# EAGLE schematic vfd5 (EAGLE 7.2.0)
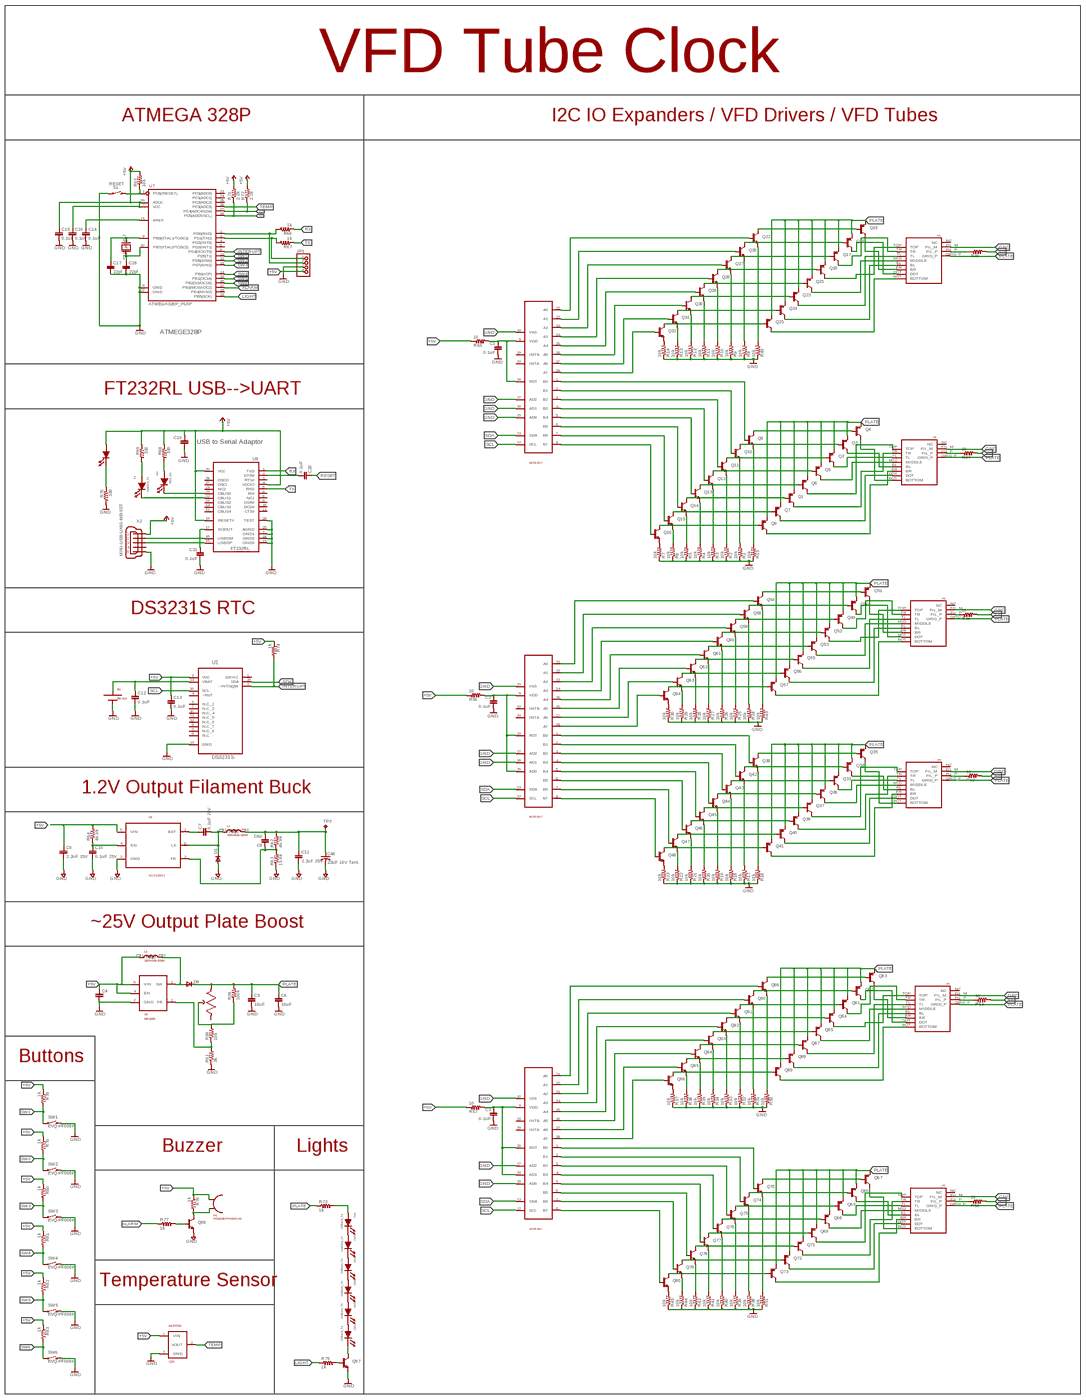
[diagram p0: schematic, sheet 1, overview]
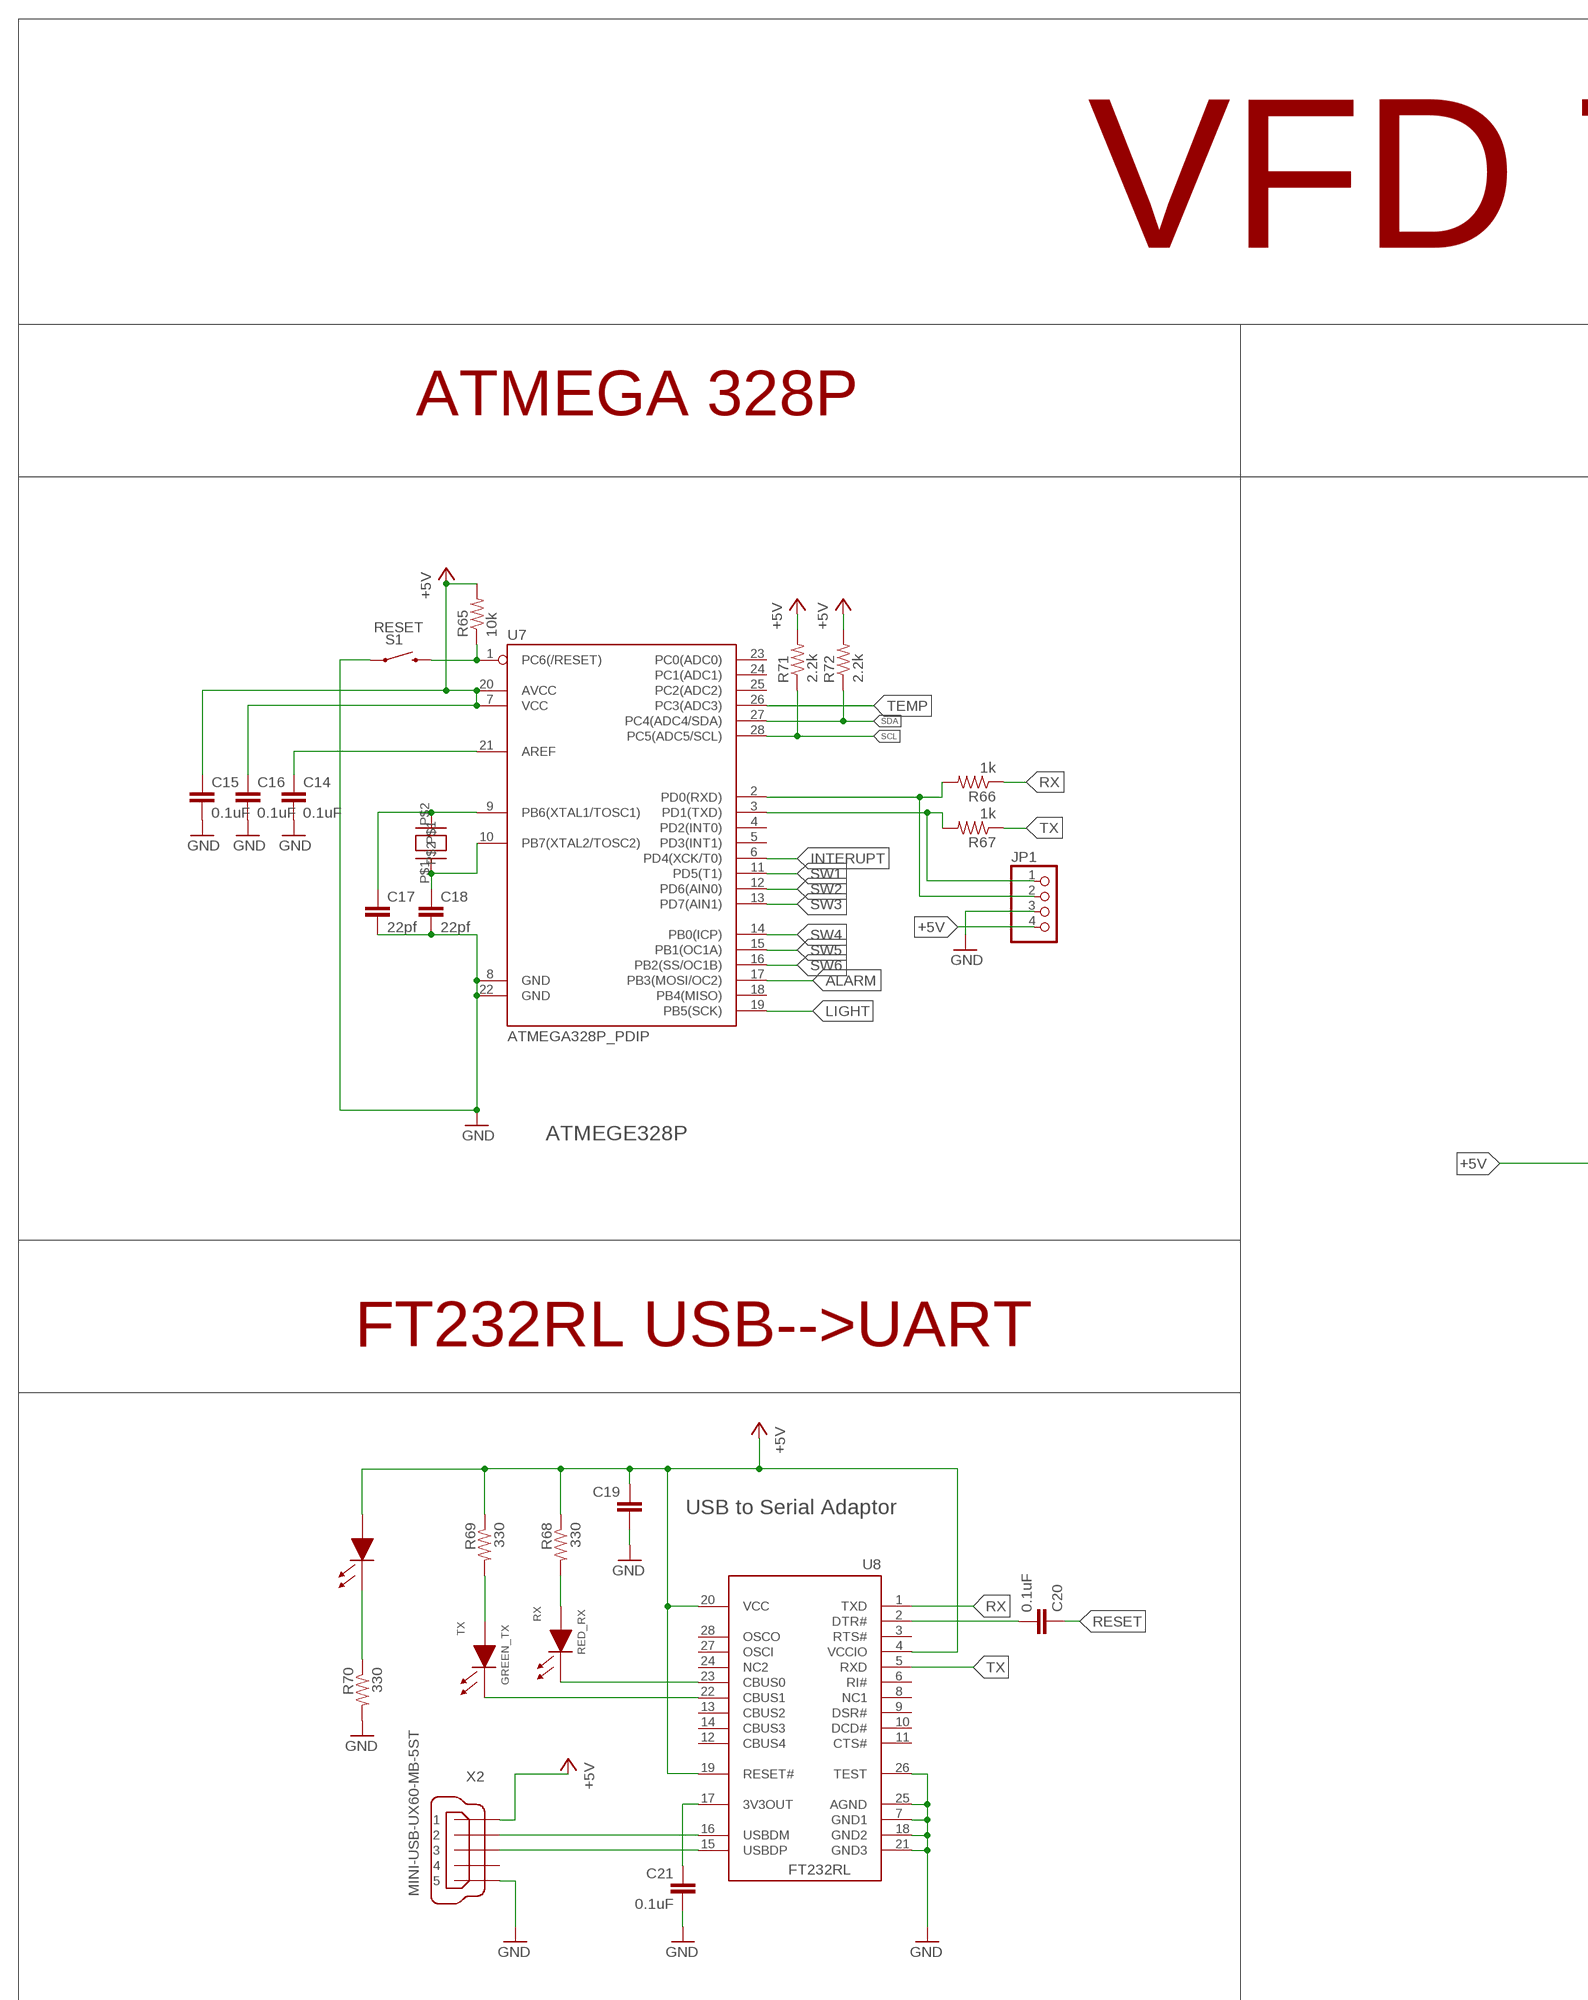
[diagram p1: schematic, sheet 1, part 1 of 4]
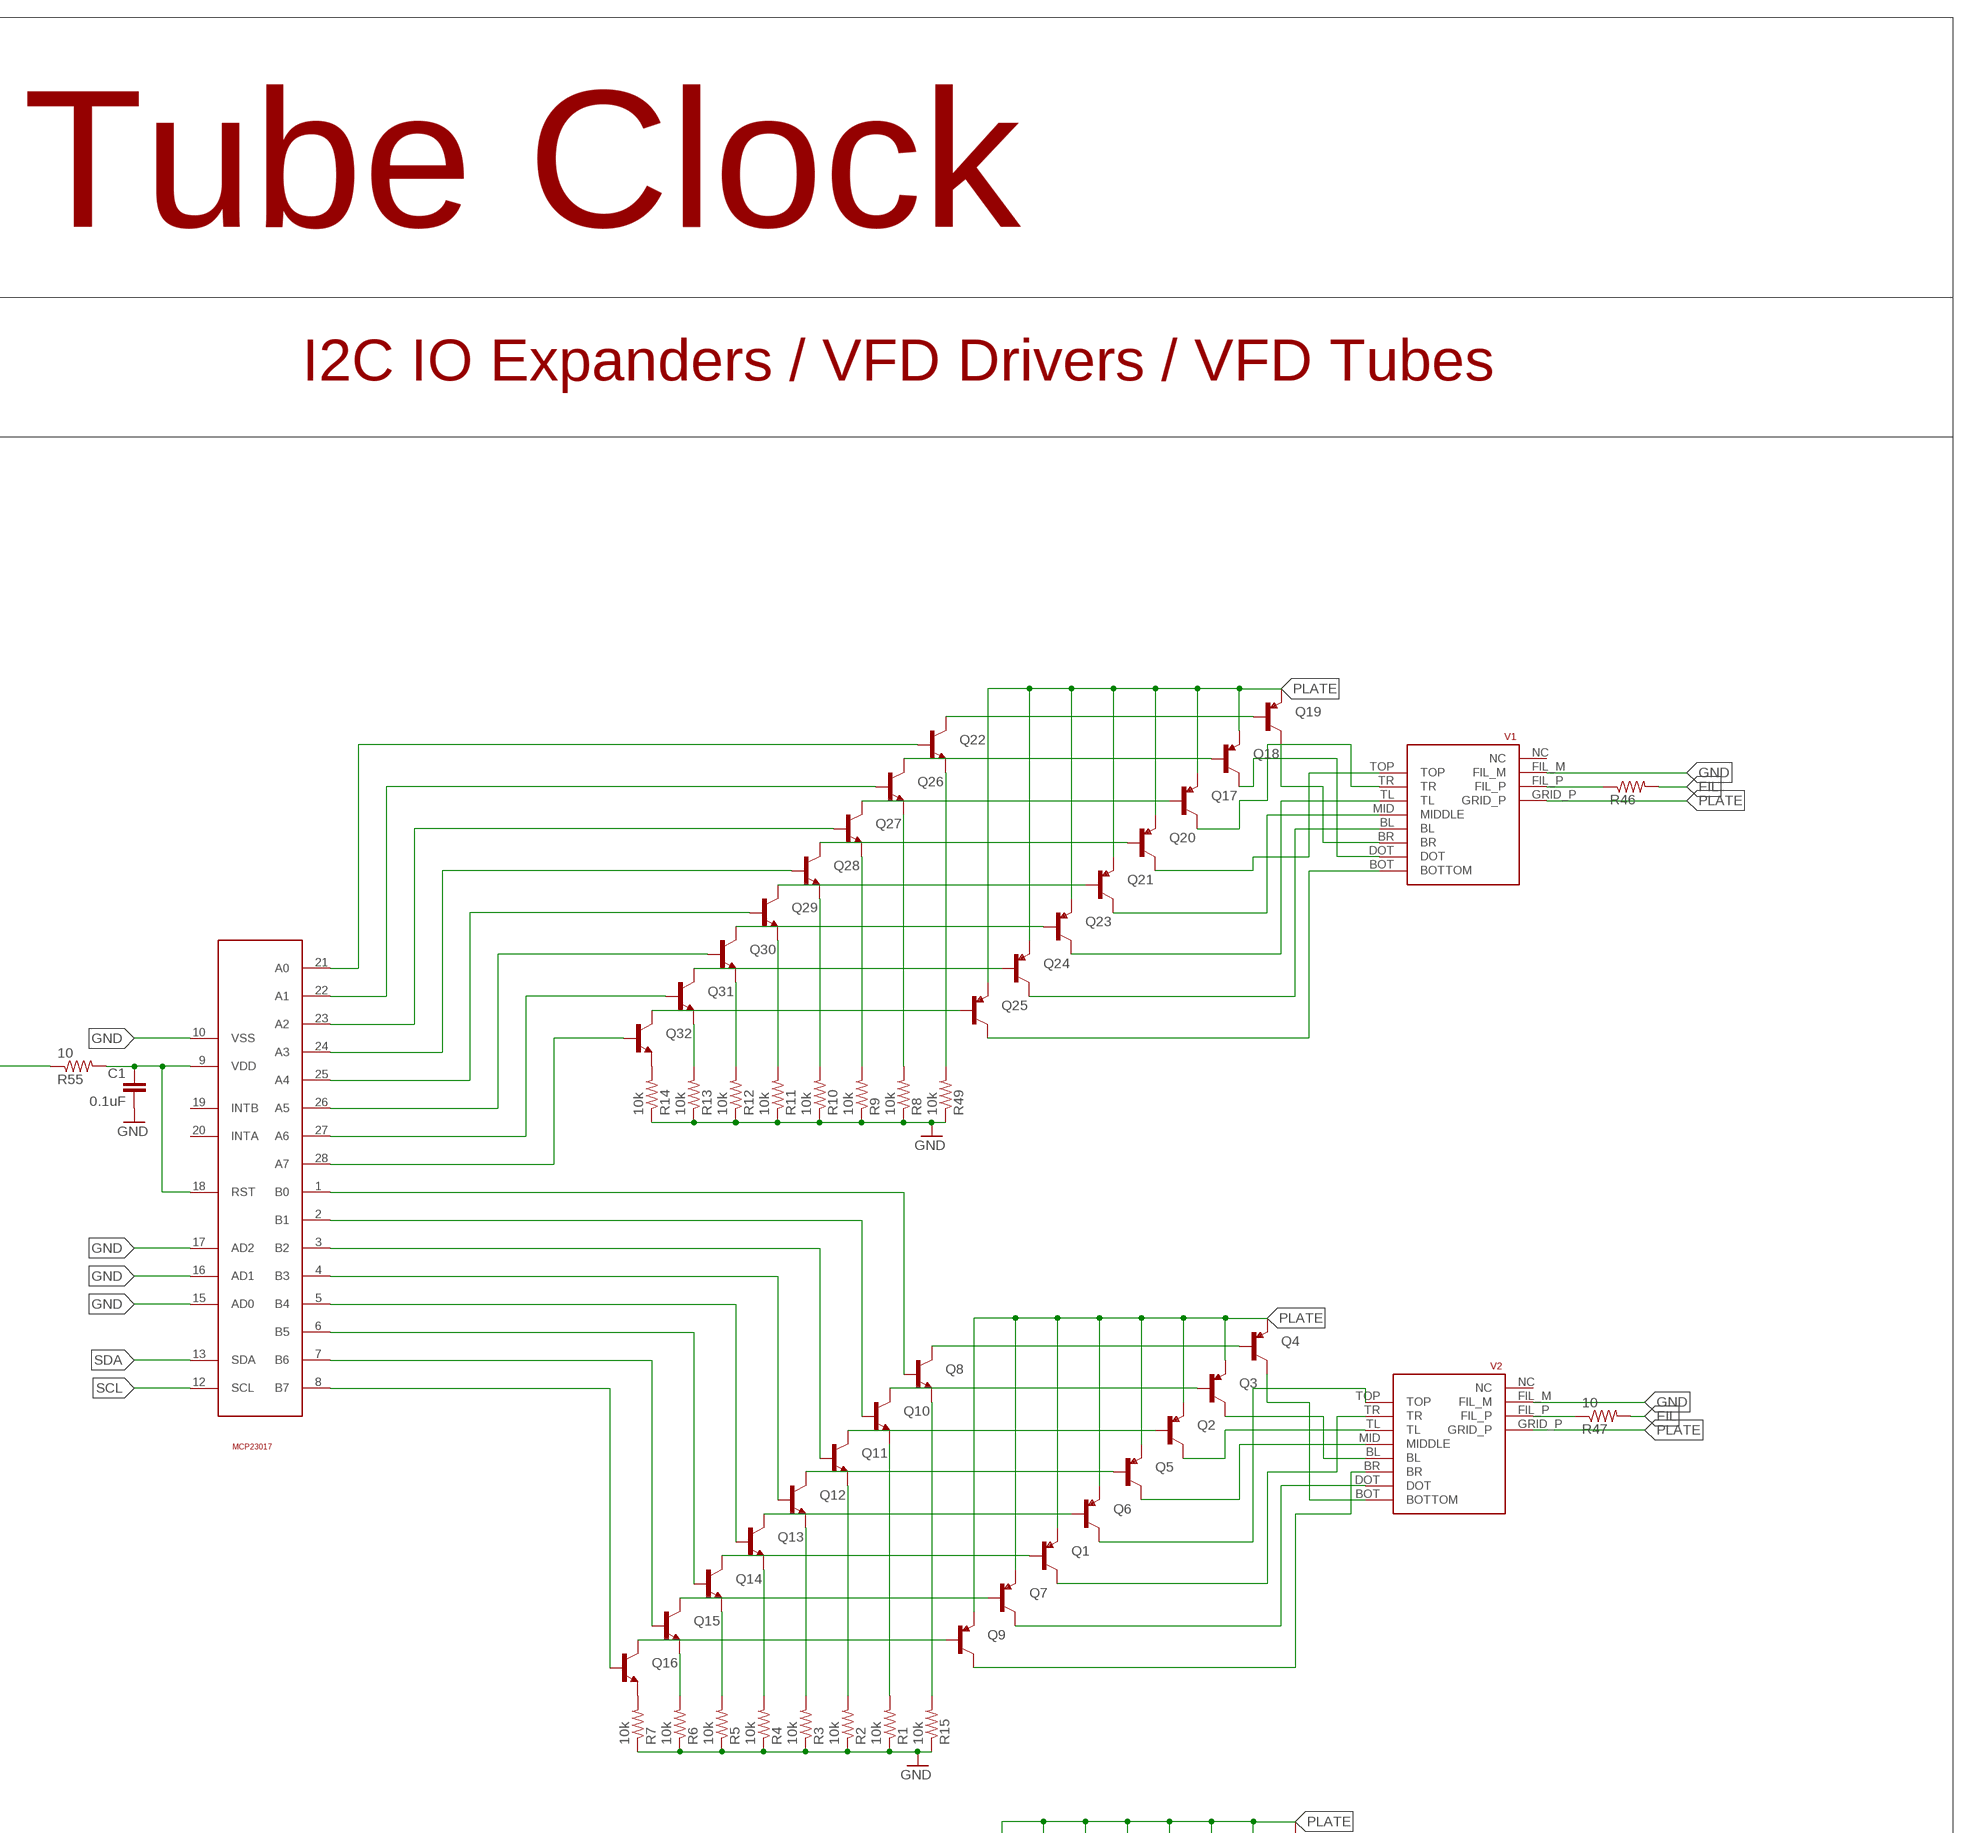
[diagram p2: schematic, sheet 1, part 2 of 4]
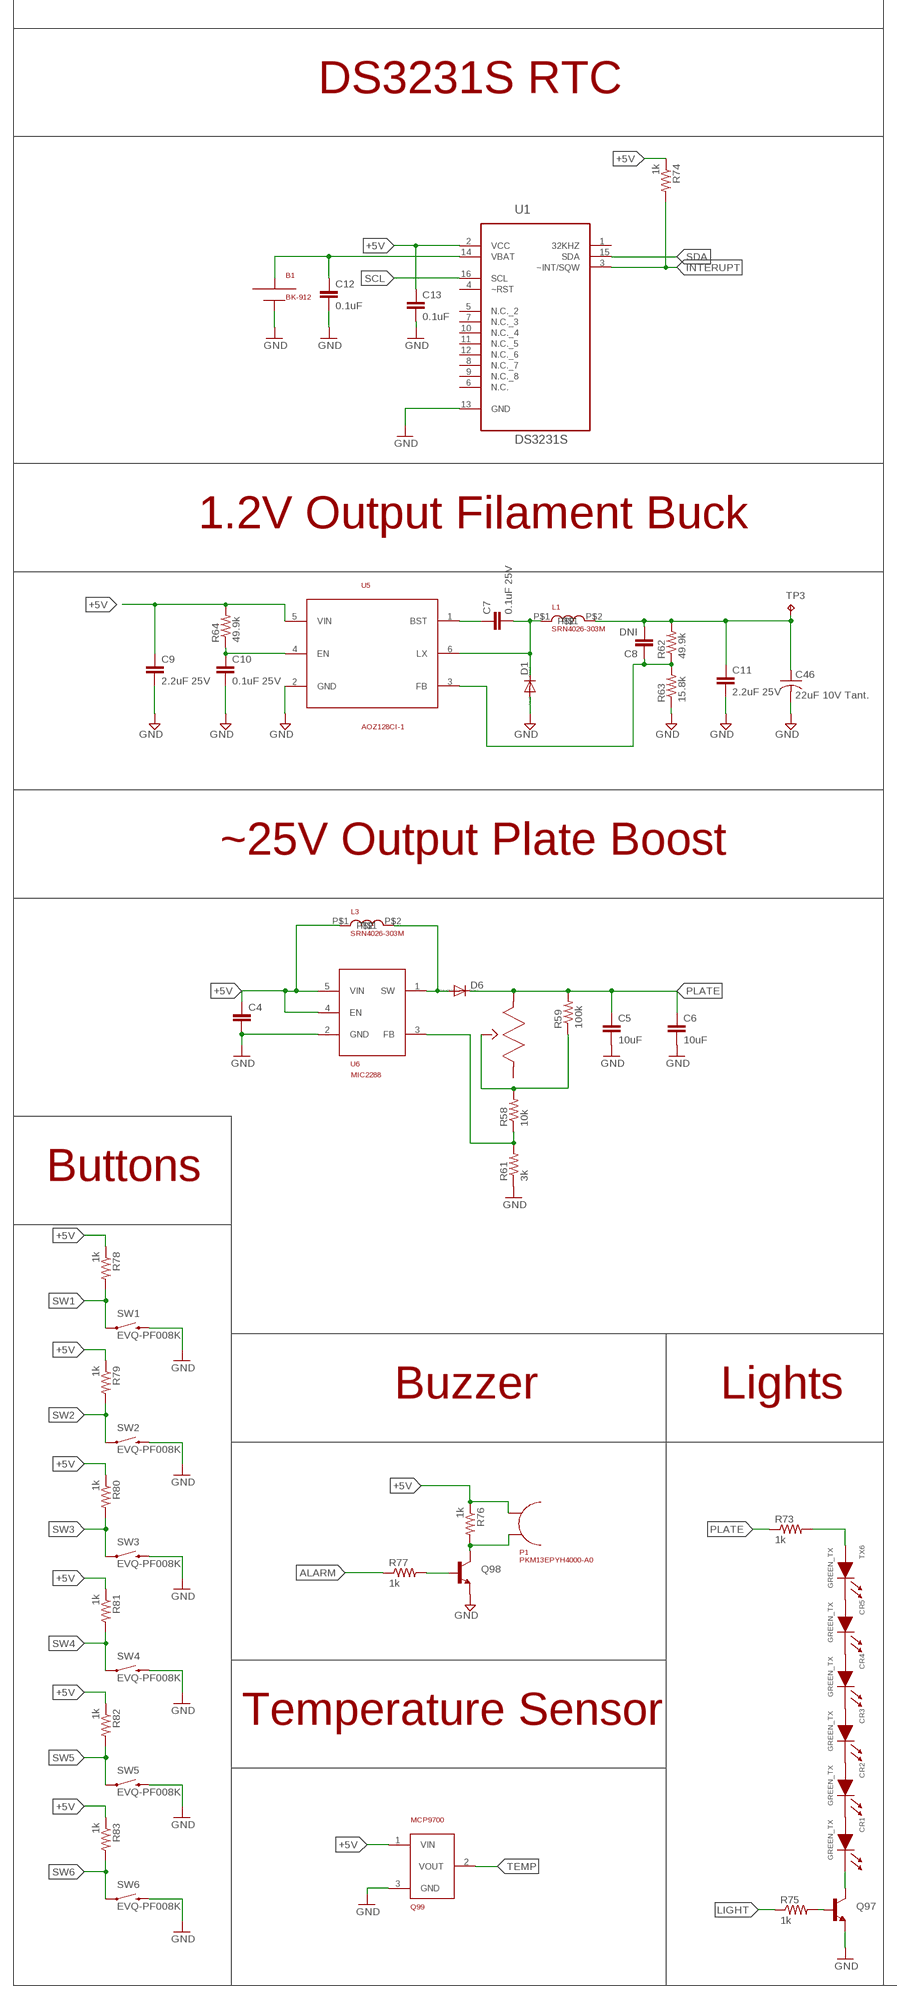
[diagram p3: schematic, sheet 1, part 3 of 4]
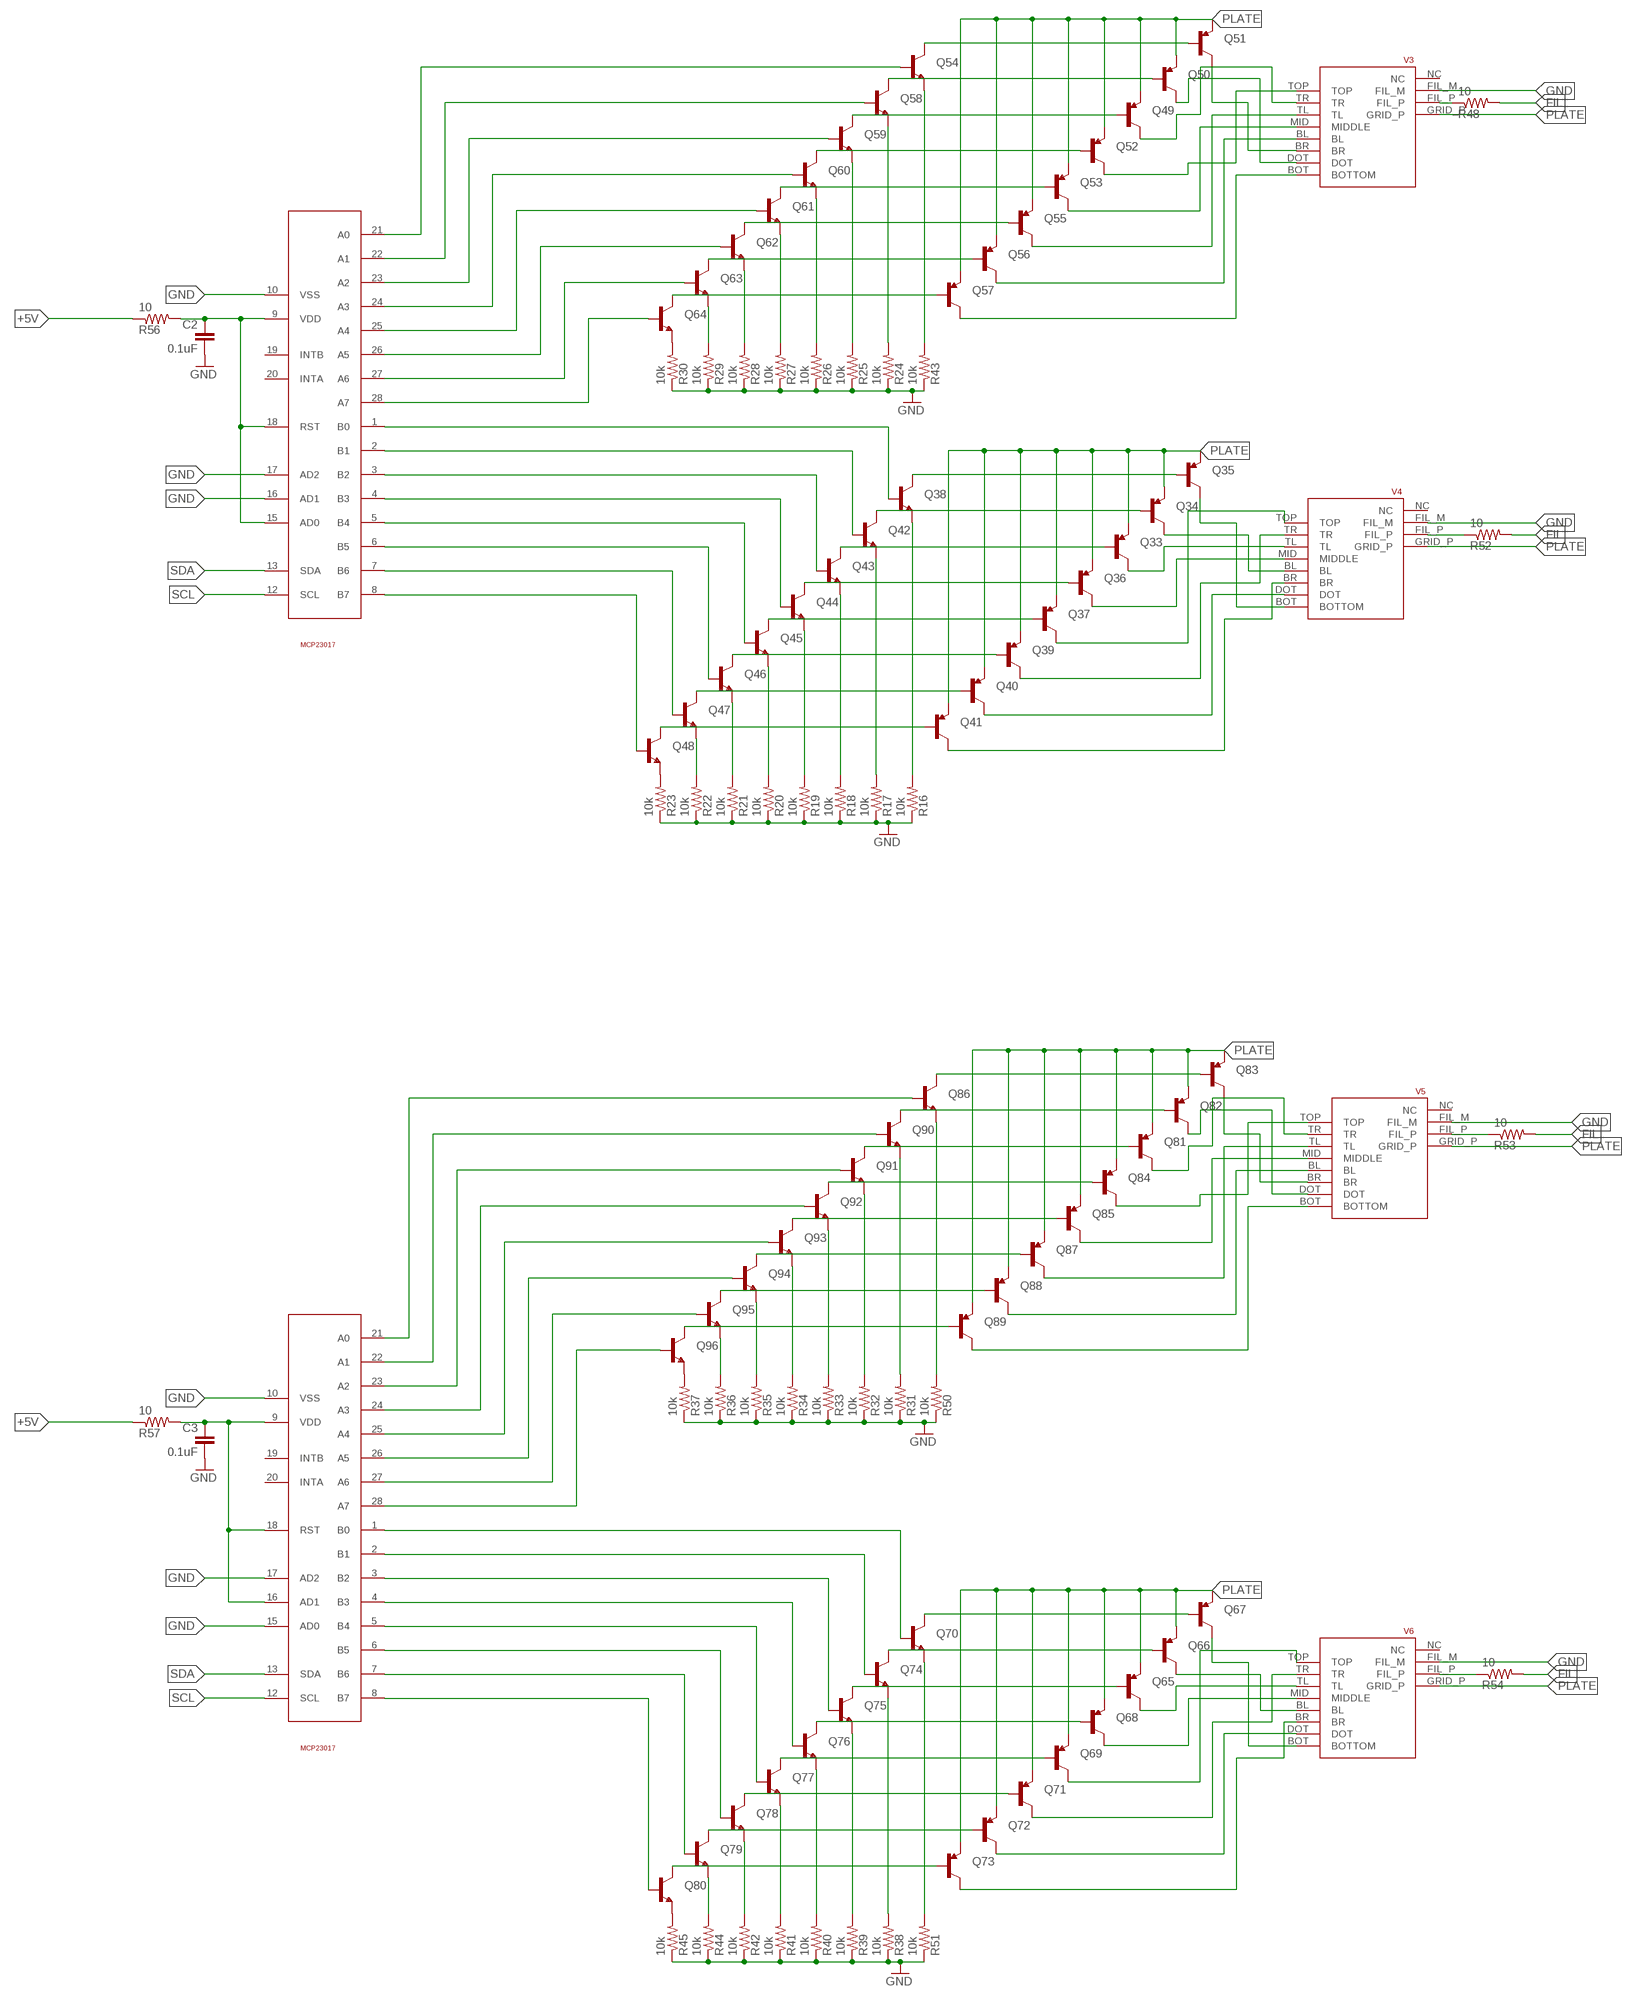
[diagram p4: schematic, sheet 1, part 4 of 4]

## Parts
B1  BK-912  [BK-912]
C1  0.1uF  C-EUC0603K  [C0603K]
C2  0.1uF  C-EUC0603K  [C0603K]
C3  0.1uF  C-EUC0603K  [C0603K]
C4  C-EUC1210  [C1210]
C5  10uF  C-EUC1210  [C1210]
C6  10uF  C-EUC1210  [C1210]
C7  0.1uF 25V  C-EUC0805  [C0805]
C8  DNI  C-EUC0805  [C0805]
C9  2.2uF 25V  C-EUC1210  [C1210]
C10  0.1uF 25V  C-EUC0805  [C0805]
C11  2.2uF 25V  C-EUC1210  [C1210]
C12  0.1uF  C-EUC0603  [C0603]
C13  0.1uF  C-EUC0603  [C0603]
C14  0.1uF  C-EUC0603  [C0603]
C15  0.1uF  C-EUC0603  [C0603]
C16  0.1uF  C-EUC0603  [C0603]
C17  22pf  CAP0805  [0805]
C18  22pf  CAP0805  [0805]
C19  C-EUC0603  [C0603]
C20  0.1uF  C-EUC0603  [C0603]
C21  0.1uF  C-EUC0603  [C0603]
C46  22uF 10V Tant.  C-USC1210  [C1210]
CR1  GREEN_TX  LED0805  [LED0805]
CR2  GREEN_TX  LED0805  [LED0805]
CR3  GREEN_TX  LED0805  [LED0805]
CR4  GREEN_TX  LED0805  [LED0805]
CR5  GREEN_TX  LED0805  [LED0805]
D1  RF081M2SCT-ND  DIODE-SOD123  [SOD123]
D6  RF081M2SCT-ND  DIODE-SOD123  [SOD123]
JP1  PINHD-1X4  [1X04]
L1  SRN4026-303M  [SRN4026]
L3  SRN4026-303M  [SRN4026]
P1  PKM13EPYH4000-A0  [PKM13EPYH4000-A0]
PWR  PWR  LED0805  [LED0805]
Q1  TRANSISTOR_PNPSMD  [SOT23-3]
Q2  TRANSISTOR_PNPSMD  [SOT23-3]
Q3  TRANSISTOR_PNPSMD  [SOT23-3]
Q4  TRANSISTOR_PNPSMD  [SOT23-3]
Q5  TRANSISTOR_PNPSMD  [SOT23-3]
Q6  TRANSISTOR_PNPSMD  [SOT23-3]
Q7  TRANSISTOR_PNPSMD  [SOT23-3]
Q8  TRANSISTOR_NPNSOT23-3  [SOT23-3]
Q9  TRANSISTOR_PNPSMD  [SOT23-3]
Q10  TRANSISTOR_NPNSOT23-3  [SOT23-3]
Q11  TRANSISTOR_NPNSOT23-3  [SOT23-3]
Q12  TRANSISTOR_NPNSOT23-3  [SOT23-3]
Q13  TRANSISTOR_NPNSOT23-3  [SOT23-3]
Q14  TRANSISTOR_NPNSOT23-3  [SOT23-3]
Q15  TRANSISTOR_NPNSOT23-3  [SOT23-3]
Q16  TRANSISTOR_NPNSOT23-3  [SOT23-3]
Q17  TRANSISTOR_PNPSMD  [SOT23-3]
Q18  TRANSISTOR_PNPSMD  [SOT23-3]
Q19  TRANSISTOR_PNPSMD  [SOT23-3]
Q20  TRANSISTOR_PNPSMD  [SOT23-3]
Q21  TRANSISTOR_PNPSMD  [SOT23-3]
Q22  TRANSISTOR_NPNSOT23-3  [SOT23-3]
Q23  TRANSISTOR_PNPSMD  [SOT23-3]
Q24  TRANSISTOR_PNPSMD  [SOT23-3]
Q25  TRANSISTOR_PNPSMD  [SOT23-3]
Q26  TRANSISTOR_NPNSOT23-3  [SOT23-3]
Q27  TRANSISTOR_NPNSOT23-3  [SOT23-3]
Q28  TRANSISTOR_NPNSOT23-3  [SOT23-3]
Q29  TRANSISTOR_NPNSOT23-3  [SOT23-3]
Q30  TRANSISTOR_NPNSOT23-3  [SOT23-3]
Q31  TRANSISTOR_NPNSOT23-3  [SOT23-3]
Q32  TRANSISTOR_NPNSOT23-3  [SOT23-3]
Q33  TRANSISTOR_PNPSMD  [SOT23-3]
Q34  TRANSISTOR_PNPSMD  [SOT23-3]
Q35  TRANSISTOR_PNPSMD  [SOT23-3]
Q36  TRANSISTOR_PNPSMD  [SOT23-3]
Q37  TRANSISTOR_PNPSMD  [SOT23-3]
Q38  TRANSISTOR_NPNSOT23-3  [SOT23-3]
Q39  TRANSISTOR_PNPSMD  [SOT23-3]
Q40  TRANSISTOR_PNPSMD  [SOT23-3]
Q41  TRANSISTOR_PNPSMD  [SOT23-3]
Q42  TRANSISTOR_NPNSOT23-3  [SOT23-3]
Q43  TRANSISTOR_NPNSOT23-3  [SOT23-3]
Q44  TRANSISTOR_NPNSOT23-3  [SOT23-3]
Q45  TRANSISTOR_NPNSOT23-3  [SOT23-3]
Q46  TRANSISTOR_NPNSOT23-3  [SOT23-3]
Q47  TRANSISTOR_NPNSOT23-3  [SOT23-3]
Q48  TRANSISTOR_NPNSOT23-3  [SOT23-3]
Q49  TRANSISTOR_PNPSMD  [SOT23-3]
Q50  TRANSISTOR_PNPSMD  [SOT23-3]
Q51  TRANSISTOR_PNPSMD  [SOT23-3]
Q52  TRANSISTOR_PNPSMD  [SOT23-3]
Q53  TRANSISTOR_PNPSMD  [SOT23-3]
Q54  TRANSISTOR_NPNSOT23-3  [SOT23-3]
Q55  TRANSISTOR_PNPSMD  [SOT23-3]
Q56  TRANSISTOR_PNPSMD  [SOT23-3]
Q57  TRANSISTOR_PNPSMD  [SOT23-3]
Q58  TRANSISTOR_NPNSOT23-3  [SOT23-3]
Q59  TRANSISTOR_NPNSOT23-3  [SOT23-3]
Q60  TRANSISTOR_NPNSOT23-3  [SOT23-3]
Q61  TRANSISTOR_NPNSOT23-3  [SOT23-3]
Q62  TRANSISTOR_NPNSOT23-3  [SOT23-3]
Q63  TRANSISTOR_NPNSOT23-3  [SOT23-3]
Q64  TRANSISTOR_NPNSOT23-3  [SOT23-3]
Q65  TRANSISTOR_PNPSMD  [SOT23-3]
Q66  TRANSISTOR_PNPSMD  [SOT23-3]
Q67  TRANSISTOR_PNPSMD  [SOT23-3]
Q68  TRANSISTOR_PNPSMD  [SOT23-3]
Q69  TRANSISTOR_PNPSMD  [SOT23-3]
Q70  TRANSISTOR_NPNSOT23-3  [SOT23-3]
Q71  TRANSISTOR_PNPSMD  [SOT23-3]
Q72  TRANSISTOR_PNPSMD  [SOT23-3]
Q73  TRANSISTOR_PNPSMD  [SOT23-3]
Q74  TRANSISTOR_NPNSOT23-3  [SOT23-3]
Q75  TRANSISTOR_NPNSOT23-3  [SOT23-3]
Q76  TRANSISTOR_NPNSOT23-3  [SOT23-3]
Q77  TRANSISTOR_NPNSOT23-3  [SOT23-3]
Q78  TRANSISTOR_NPNSOT23-3  [SOT23-3]
Q79  TRANSISTOR_NPNSOT23-3  [SOT23-3]
Q80  TRANSISTOR_NPNSOT23-3  [SOT23-3]
Q81  TRANSISTOR_PNPSMD  [SOT23-3]
Q82  TRANSISTOR_PNPSMD  [SOT23-3]
Q83  TRANSISTOR_PNPSMD  [SOT23-3]
Q84  TRANSISTOR_PNPSMD  [SOT23-3]
Q85  TRANSISTOR_PNPSMD  [SOT23-3]
Q86  TRANSISTOR_NPNSOT23-3  [SOT23-3]
Q87  TRANSISTOR_PNPSMD  [SOT23-3]
Q88  TRANSISTOR_PNPSMD  [SOT23-3]
Q89  TRANSISTOR_PNPSMD  [SOT23-3]
Q90  TRANSISTOR_NPNSOT23-3  [SOT23-3]
Q91  TRANSISTOR_NPNSOT23-3  [SOT23-3]
Q92  TRANSISTOR_NPNSOT23-3  [SOT23-3]
Q93  TRANSISTOR_NPNSOT23-3  [SOT23-3]
Q94  TRANSISTOR_NPNSOT23-3  [SOT23-3]
Q95  TRANSISTOR_NPNSOT23-3  [SOT23-3]
Q96  TRANSISTOR_NPNSOT23-3  [SOT23-3]
Q97  TRANSISTOR_NPNSOT23-3  [SOT23-3]
Q98  TRANSISTOR_NPNSOT23-3  [SOT23-3]
Q99  MCP9700  [SOT23-3]
R1  10k  R-US_R0603  [R0603]
R2  10k  R-US_R0603  [R0603]
R3  10k  R-US_R0603  [R0603]
R4  10k  R-US_R0603  [R0603]
R5  10k  R-US_R0603  [R0603]
R6  10k  R-US_R0603  [R0603]
R7  10k  R-US_R0603  [R0603]
R8  10k  R-US_R0603  [R0603]
R9  10k  R-US_R0603  [R0603]
R10  10k  R-US_R0603  [R0603]
R11  10k  R-US_R0603  [R0603]
R12  10k  R-US_R0603  [R0603]
R13  10k  R-US_R0603  [R0603]
R14  10k  R-US_R0603  [R0603]
R15  10k  R-US_R0603  [R0603]
R16  10k  R-US_R0603  [R0603]
R17  10k  R-US_R0603  [R0603]
R18  10k  R-US_R0603  [R0603]
R19  10k  R-US_R0603  [R0603]
R20  10k  R-US_R0603  [R0603]
R21  10k  R-US_R0603  [R0603]
R22  10k  R-US_R0603  [R0603]
R23  10k  R-US_R0603  [R0603]
R24  10k  R-US_R0603  [R0603]
R25  10k  R-US_R0603  [R0603]
R26  10k  R-US_R0603  [R0603]
R27  10k  R-US_R0603  [R0603]
R28  10k  R-US_R0603  [R0603]
R29  10k  R-US_R0603  [R0603]
R30  10k  R-US_R0603  [R0603]
R31  10k  R-US_R0603  [R0603]
R32  10k  R-US_R0603  [R0603]
R33  10k  R-US_R0603  [R0603]
R34  10k  R-US_R0603  [R0603]
R35  10k  R-US_R0603  [R0603]
R36  10k  R-US_R0603  [R0603]
R37  10k  R-US_R0603  [R0603]
R38  10k  R-US_R0603  [R0603]
R39  10k  R-US_R0603  [R0603]
R40  10k  R-US_R0603  [R0603]
R41  10k  R-US_R0603  [R0603]
R42  10k  R-US_R0603  [R0603]
R43  10k  R-US_R0603  [R0603]
R44  10k  R-US_R0603  [R0603]
R45  10k  R-US_R0603  [R0603]
R46  R-US_R0603  [R0603]
R47  10  R-US_R0603  [R0603]
R48  10  R-US_R0603  [R0603]
R49  10k  R-US_R0603  [R0603]
R50  10k  R-US_R0603  [R0603]
R51  10k  R-US_R0603  [R0603]
R52  10  R-US_R0603  [R0603]
R53  10  R-US_R0603  [R0603]
R54  10  R-US_R0603  [R0603]
R55  10  R-US_R0603  [R0603]
R56  10  R-US_R0603  [R0603]
R57  10  R-US_R0603  [R0603]
R58  10k  R-US_R0603  [R0603]
R59  100k  R-US_R0603  [R0603]
R61  3k  R-US_R0603  [R0603]
R62  49.9k  R-US_R0603  [R0603]
R63  15.8k  R-US_R0603  [R0603]
R64  49.9k  R-US_R0603  [R0603]
R65  10k  RESISTOR0805-RES  [0805]
R66  1k  RESISTOR0805-RES  [0805]
R67  1k  RESISTOR0805-RES  [0805]
R68  330  RESISTOR0805-RES  [0805]
R69  330  RESISTOR0805-RES  [0805]
R70  330  RESISTOR0805-RES  [0805]
R71  2.2k  RESISTOR0805-RES  [0805]
R72  2.2k  RESISTOR0805-RES  [0805]
R73  1k  RESISTOR0805-RES  [0805]
R74  1k  R-US_R0603  [R0603]
R75  1k  RESISTOR0805-RES  [0805]
R76  1k  RESISTOR0805-RES  [0805]
R77  1k  RESISTOR0805-RES  [0805]
R78  1k  R-US_R0603  [R0603]
R79  1k  R-US_R0603  [R0603]
R80  1k  R-US_R0603  [R0603]
R81  1k  R-US_R0603  [R0603]
R82  1k  R-US_R0603  [R0603]
R83  1k  R-US_R0603  [R0603]
R100  3224G-1-104E  [3224G]
RX  RED_RX  LED0805  [LED0805]
S1  SWITCH-MOMENTARY-2PTH  [TACTILE-PTH]
SW1  EVQ-PF008K  [EVQ-PF008K]
SW2  EVQ-PF008K  [EVQ-PF008K]
SW3  EVQ-PF008K  [EVQ-PF008K]
SW4  EVQ-PF008K  [EVQ-PF008K]
SW5  EVQ-PF008K  [EVQ-PF008K]
SW6  EVQ-PF008K  [EVQ-PF008K]
TP3  TPPAD1-13  [P1-13]
TX  GREEN_TX  LED0805  [LED0805]
TX6  GREEN_TX  LED0805  [LED0805]
U1  DS3231S  [SOIC127P1032X265-16N]
U2  MCP23017  [SSOP16]
U3  MCP23017  [SSOP16]
U4  MCP23017  [SSOP16]
U5  AOZ128CI-1  [SOT236]
U6  MIC2288  [SOT23-5]
U7  ATMEGA328P_PDIP  [DIL28-3]
U8  FT232RL  [SSOP28]
V1  IV6_NUMITRON  [IV6_NUMITRON_PAC]
V2  IV6_NUMITRON  [IV6_NUMITRON_PAC]
V3  IV6_NUMITRON  [IV6_NUMITRON_PAC]
V4  IV6_NUMITRON  [IV6_NUMITRON_PAC]
V5  IV6_NUMITRON  [IV6_NUMITRON_PAC]
V6  IV6_NUMITRON  [IV6_NUMITRON_PAC]
X2  MINI-USB-UX60-MB-5ST  [UX60-MB-5ST]
X3  ECS-80-20  [CSM7X]

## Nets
+5V: C4.1 C9.1 C13.1 C15.1 C16.1 C19.1 JP1.4 L3.P$1 P1.P$1 PWR.2(AN) Q99.1(VIN) R55.1 R56.1 R57.1 R64.2 R65.2 R68.1 R69.1 R71.2 R72.2 R74.1 R76.1 R78.1 R79.1 R80.1 R81.1 R82.1 R83.1 U1.2(VCC) U5.5(VIN) U6.4(EN) U6.5(VIN) U7.7(VCC) U7.20(AVCC) U8.4(VCCIO) U8.19(RESET#) U8.20(VCC) X2.1
ALARM: R77.1 U7.17(PB3(MOSI/OC2))
FIL: C8.2 C11.1 C46.1 L1.P$2 R46.2 R47.2 R48.2 R52.2 R53.2 R54.2 R62.2 TP3.TP
GND: B1.- C1.2 C2.2 C3.2 C4.2 C5.2 C6.2 C9.2 C10.2 C11.2 C12.2 C13.2 C14.2 C15.2 C16.2 C17.2 C18.2 C19.2 C21.2 C46.2 D1.A JP1.3 Q97.2(E) Q98.2(E) Q99.3(GND) R1.1 R2.1 R3.1 R4.1 R5.1 R6.1 R7.1 R8.1 R9.1 R10.1 R11.1 R12.1 R13.1 R14.1 R15.1 R16.1 R17.1 R18.1 R19.1 R20.1 R21.1 R22.1 R23.1 R24.1 R25.1 R26.1 R27.1 R28.1 R29.1 R30.1 R31.1 R32.1 R33.1 R34.1 R35.1 R36.1 R37.1 R38.1 R39.1 R40.1 R41.1 R42.1 R43.1 R44.1 R45.1 R49.1 R50.1 R51.1 R61.1 R63.1 R70.2 S1.1 SW1.S2 SW2.S2 SW3.S2 SW4.S2 SW5.S2 SW6.S2 U1.13(GND) U2.10(VSS) U2.15(AD0) U2.16(AD1) U2.17(AD2) U3.10(VSS) U3.16(AD1) U3.17(AD2) U4.10(VSS) U4.15(AD0) U4.17(AD2) U5.2(GND) U6.2(GND) U7.8(GND) U7.22(GND) U8.7(GND1) U8.18(GND2) U8.21(GND3) U8.25(AGND) U8.26(TEST) V1.FIL_M V2.FIL_M V3.FIL_M V4.FIL_M V5.FIL_M V6.FIL_M X2.5
INTERUPT: R74.2 U1.3(~INT/SQW) U7.6(PD4(XCK/T0))
LIGHT: R75.1 U7.19(PB5(SCK))
N$1: Q35.3(C) V4.BOT(BOTTOM)
N$2: Q22.1(B) U2.21(A0)
N$3: Q17.3(C) V1.TR
N$4: Q4.3(C) V2.BOT(BOTTOM)
N$5: Q32.2(E) R14.2
N$6: Q3.3(C) V2.BL
N$7: Q2.3(C) V2.TL
N$8: Q5.3(C) V2.MID(MIDDLE)
N$9: Q6.3(C) V2.TOP
N$10: Q1.3(C) V2.TR
N$11: Q7.3(C) V2.DOT
N$12: Q26.1(B) U2.22(A1)
N$13: Q9.3(C) V2.BR
N$14: Q4.1(B) Q8.3(C)
N$15: Q3.1(B) Q10.3(C)
N$16: Q2.1(B) Q11.3(C)
N$17: Q5.1(B) Q12.3(C)
N$18: Q6.1(B) Q13.3(C)
N$19: Q1.1(B) Q14.3(C)
N$20: Q7.1(B) Q15.3(C)
N$21: Q18.3(C) V1.DOT
N$22: Q9.1(B) Q16.3(C)
N$23: Q11.2(E) R2.2
N$24: Q12.2(E) R3.2
N$25: Q8.2(E) R15.2
N$26: Q13.2(E) R4.2
N$27: Q16.2(E) R7.2
N$28: Q14.2(E) R5.2
N$29: Q15.2(E) R6.2
N$30: Q10.2(E) R1.2
N$31: Q8.1(B) U2.1(B0)
N$32: Q10.1(B) U2.2(B1)
N$33: Q11.1(B) U2.3(B2)
N$34: Q12.1(B) U2.4(B3)
N$35: Q13.1(B) U2.5(B4)
N$36: Q14.1(B) U2.6(B5)
N$37: Q15.1(B) U2.7(B6)
N$38: Q16.1(B) U2.8(B7)
N$39: Q21.3(C) V1.MID(MIDDLE)
N$40: Q23.3(C) V1.TL
N$41: Q24.3(C) V1.BL
N$42: Q25.3(C) V1.BOT(BOTTOM)
N$43: Q19.1(B) Q22.3(C)
N$44: Q18.1(B) Q26.3(C)
N$45: Q17.1(B) Q27.3(C)
N$46: Q20.1(B) Q28.3(C)
N$47: Q21.1(B) Q29.3(C)
N$48: Q23.1(B) Q30.3(C)
N$49: Q24.1(B) Q31.3(C)
N$50: Q25.1(B) Q32.3(C)
N$51: Q64.2(E) R30.2
N$52: Q27.2(E) R9.2
N$53: Q28.2(E) R10.2
N$54: Q29.2(E) R11.2
N$55: Q30.2(E) R12.2
N$56: Q48.2(E) R23.2
N$57: R47.1 V2.FIL_P
N$58: Q31.2(E) R13.2
N$59: Q26.2(E) R8.2
N$60: Q27.1(B) U2.23(A2)
N$61: Q28.1(B) U2.24(A3)
N$62: Q29.1(B) U2.25(A4)
N$63: Q30.1(B) U2.26(A5)
N$64: Q31.1(B) U2.27(A6)
N$65: Q32.1(B) U2.28(A7)
N$66: Q54.1(B) U3.21(A0)
N$67: Q58.1(B) U3.22(A1)
N$68: Q59.1(B) U3.23(A2)
N$69: Q60.1(B) U3.24(A3)
N$70: Q22.2(E) R49.2
N$71: Q61.1(B) U3.25(A4)
N$72: C1.1 R55.2 U2.9(VDD) U2.18(RST)
N$73: C2.1 R56.2 U3.9(VDD) U3.15(AD0) U3.18(RST)
N$74: C3.1 R57.2 U4.9(VDD) U4.16(AD1) U4.18(RST)
N$75: Q62.1(B) U3.26(A5)
N$76: Q96.2(E) R37.2
N$77: Q19.3(C) V1.BR
N$78: Q33.3(C) V4.TL
N$79: Q20.3(C) V1.TOP
N$80: Q36.3(C) V4.MID(MIDDLE)
N$81: Q37.3(C) V4.TOP
N$82: Q39.3(C) V4.TR
N$83: Q40.3(C) V4.DOT
N$84: Q41.3(C) V4.BR
N$85: Q35.1(B) Q38.3(C)
N$86: Q34.1(B) Q42.3(C)
N$87: Q33.1(B) Q43.3(C)
N$88: Q80.2(E) R45.2
N$89: Q36.1(B) Q44.3(C)
N$90: Q37.1(B) Q45.3(C)
N$91: Q39.1(B) Q46.3(C)
N$92: Q40.1(B) Q47.3(C)
N$93: Q41.1(B) Q48.3(C)
N$94: Q63.1(B) U3.27(A6)
N$95: Q43.2(E) R18.2
N$96: Q44.2(E) R19.2
N$97: Q45.2(E) R20.2
N$98: Q46.2(E) R21.2
N$99: Q47.2(E) R22.2
N$100: Q42.2(E) R17.2
N$101: Q64.1(B) U3.28(A7)
N$102: Q38.1(B) U3.1(B0)
N$103: Q42.1(B) U3.2(B1)
N$104: Q43.1(B) U3.3(B2)
N$105: Q44.1(B) U3.4(B3)
N$106: Q45.1(B) U3.5(B4)
N$107: Q46.1(B) U3.6(B5)
N$108: Q47.1(B) U3.7(B6)
N$109: Q48.1(B) U3.8(B7)
N$110: Q86.1(B) U4.21(A0)
N$111: Q38.2(E) R16.2
N$112: Q34.3(C) V4.BL
N$113: C7.1 U5.1(BST)
N$114: Q90.1(B) U4.22(A1)
N$115: Q91.1(B) U4.23(A2)
N$116: Q92.1(B) U4.24(A3)
N$117: Q93.1(B) U4.25(A4)
N$118: Q94.1(B) U4.26(A5)
N$119: Q49.3(C) V3.TR
N$120: Q53.3(C) V3.MID(MIDDLE)
N$121: Q95.1(B) U4.27(A6)
N$122: Q55.3(C) V3.TL
N$123: Q56.3(C) V3.BL
N$124: Q57.3(C) V3.BOT(BOTTOM)
N$125: Q51.1(B) Q54.3(C)
N$126: Q50.1(B) Q58.3(C)
N$127: Q49.1(B) Q59.3(C)
N$128: Q52.1(B) Q60.3(C)
N$129: Q53.1(B) Q61.3(C)
N$130: Q55.1(B) Q62.3(C)
N$131: Q56.1(B) Q63.3(C)
N$132: Q57.1(B) Q64.3(C)
N$133: Q96.1(B) U4.28(A7)
N$134: Q59.2(E) R25.2
N$135: Q60.2(E) R26.2
N$136: Q61.2(E) R27.2
N$137: Q62.2(E) R28.2
N$138: Q63.2(E) R29.2
N$139: Q58.2(E) R24.2
N$140: Q70.1(B) U4.1(B0)
N$141: R53.1 V5.FIL_P
N$142: B1.+1(+) B1.+2(+) C12.1 U1.14(VBAT)
N$143: R48.1 V3.FIL_P
N$144: R46.1 V1.FIL_P
N$145: C8.1 R62.1 R63.2 U5.3(FB)
N$146: R58.2 R59.1 R100.2
N$147: R58.1 R61.2 U6.3(FB)
N$148: C10.1 R64.1 U5.4(EN)
N$149: C17.1 U7.9(PB6(XTAL1/TOSC1)) X3.P$2
N$150: Q54.2(E) R43.2
N$151: R52.1 V4.FIL_P
N$152: R54.1 V6.FIL_P
N$153: C18.1 U7.10(PB7(XTAL2/TOSC2)) X3.P$1
N$154: C20.2 U8.2(DTR#)
N$155: U8.15(USBDP) X2.3
N$156: Q51.3(C) V3.BR
N$157: Q52.3(C) V3.TOP
N$158: Q50.3(C) V3.DOT
N$159: Q67.3(C) V6.BOT(BOTTOM)
N$160: U8.16(USBDM) X2.2
N$161: Q65.3(C) V6.TL
N$162: Q68.3(C) V6.MID(MIDDLE)
N$163: Q69.3(C) V6.TOP
N$164: Q71.3(C) V6.TR
N$165: Q72.3(C) V6.DOT
N$166: Q73.3(C) V6.BR
N$167: Q67.1(B) Q70.3(C)
N$168: Q66.1(B) Q74.3(C)
N$169: Q65.1(B) Q75.3(C)
N$170: Q68.1(B) Q76.3(C)
N$171: Q69.1(B) Q77.3(C)
N$172: Q71.1(B) Q78.3(C)
N$173: Q72.1(B) Q79.3(C)
N$174: Q73.1(B) Q80.3(C)
N$175: RX.1(CA) U8.23(CBUS0)
N$176: Q75.2(E) R39.2
N$177: Q76.2(E) R40.2
N$178: Q77.2(E) R41.2
N$179: Q78.2(E) R42.2
N$180: Q79.2(E) R44.2
N$181: Q74.2(E) R38.2
N$182: Q74.1(B) U4.2(B1)
N$183: Q75.1(B) U4.3(B2)
N$184: Q76.1(B) U4.4(B3)
N$185: Q77.1(B) U4.5(B4)
N$186: Q78.1(B) U4.6(B5)
N$187: Q79.1(B) U4.7(B6)
N$188: Q80.1(B) U4.8(B7)
N$189: TX.1(CA) U8.22(CBUS1)
N$190: C14.1 U7.21(AREF)
N$191: CR1.2(AN) CR2.1(CA)
N$192: Q70.2(E) R51.2
N$193: Q66.3(C) V6.BL
N$194: PWR.1(CA) R70.1
N$195: R68.2 RX.2(AN)
N$196: R69.2 TX.2(AN)
N$197: CR2.2(AN) CR3.1(CA)
N$198: CR3.2(AN) CR4.1(CA)
N$199: JP1.2 R66.2 U7.2(PD0(RXD))
N$200: Q81.3(C) V5.TR
N$201: Q85.3(C) V5.MID(MIDDLE)
N$202: Q87.3(C) V5.TL
N$203: Q88.3(C) V5.BL
N$204: Q89.3(C) V5.BOT(BOTTOM)
N$205: Q83.1(B) Q86.3(C)
N$206: Q82.1(B) Q90.3(C)
N$207: Q81.1(B) Q91.3(C)
N$208: Q84.1(B) Q92.3(C)
N$209: Q85.1(B) Q93.3(C)
N$210: Q87.1(B) Q94.3(C)
N$211: Q88.1(B) Q95.3(C)
N$212: Q89.1(B) Q96.3(C)
N$213: CR4.2(AN) CR5.1(CA)
N$214: Q91.2(E) R32.2
N$215: Q92.2(E) R33.2
N$216: Q93.2(E) R34.2
N$217: Q94.2(E) R35.2
N$218: Q95.2(E) R36.2
N$219: Q90.2(E) R31.2
N$220: JP1.1 R67.2 U7.3(PD1(TXD))
N$221: CR5.2(AN) TX6.1(CA)
N$222: R73.2 TX6.2(AN)
N$223: CR1.1(CA) Q97.3(C)
N$224: Q97.1(B) R75.2
N$225: P1.P$2 Q98.3(C) R76.2
N$226: Q98.1(B) R77.2
N$228: C21.1 U8.17(3V3OUT)
N$231: Q86.2(E) R50.2
N$238: Q83.3(C) V5.BR
N$239: Q84.3(C) V5.TOP
N$240: Q82.3(C) V5.DOT
PLATE: C5.1 C6.1 D6.C Q1.2(E) Q2.2(E) Q3.2(E) Q4.2(E) Q5.2(E) Q6.2(E) Q7.2(E) Q9.2(E) Q17.2(E) Q18.2(E) Q19.2(E) Q20.2(E) Q21.2(E) Q23.2(E) Q24.2(E) Q25.2(E) Q33.2(E) Q34.2(E) Q35.2(E) Q36.2(E) Q37.2(E) Q39.2(E) Q40.2(E) Q41.2(E) Q49.2(E) Q50.2(E) Q51.2(E) Q52.2(E) Q53.2(E) Q55.2(E) Q56.2(E) Q57.2(E) Q65.2(E) Q66.2(E) Q67.2(E) Q68.2(E) Q69.2(E) Q71.2(E) Q72.2(E) Q73.2(E) Q81.2(E) Q82.2(E) Q83.2(E) Q84.2(E) Q85.2(E) Q87.2(E) Q88.2(E) Q89.2(E) R59.2 R73.1 R100.1 V1.GRID_P V2.GRID_P V3.GRID_P V4.GRID_P V5.GRID_P V6.GRID_P
RESET: C20.1 R65.1 S1.3 U7.1(PC6(/RESET))
RX: R66.1 U8.1(TXD)
SCL: R71.1 U1.16(SCL) U2.12(SCL) U3.12(SCL) U4.12(SCL) U7.28(PC5(ADC5/SCL))
SDA: R72.1 U1.15(SDA) U2.13(SDA) U3.13(SDA) U4.13(SDA) U7.27(PC4(ADC4/SDA))
SW1: R78.2 SW1.S1 U7.11(PD5(T1))
SW2: R79.2 SW2.S1 U7.12(PD6(AIN0))
SW3: R80.2 SW3.S1 U7.13(PD7(AIN1))
SW4: R81.2 SW4.S1 U7.14(PB0(ICP))
SW5: R82.2 SW5.S1 U7.15(PB1(OC1A))
SW6: R83.2 SW6.S1 U7.16(PB2(SS/OC1B))
TEMP: Q99.2(VOUT) U7.26(PC3(ADC3))
TX: R67.1 U8.5(RXD)
VS5: D6.A L3.P$2 U6.1(SW)
VSW3: C7.2 D1.C L1.P$1 U5.6(LX)
Unconnected: R100.3 U1.1(32KHZ) U1.4(~RST) U1.5(N.C._2) U1.6(N.C.) U1.7(N.C._3) U1.8(N.C._7) U1.9(N.C._8) U1.10(N.C._4) U1.11(N.C._5) U1.12(N.C._6) U2.19(INTB) U2.20(INTA) U3.19(INTB) U3.20(INTA) U4.19(INTB) U4.20(INTA) U7.4(PD2(INT0)) U7.5(PD3(INT1)) U7.18(PB4(MISO)) U7.23(PC0(ADC0)) U7.24(PC1(ADC1)) U7.25(PC2(ADC2)) U8.3(RTS#) U8.6(RI#) U8.8(NC1) U8.9(DSR#) U8.10(DCD#) U8.11(CTS#) U8.12(CBUS4) U8.13(CBUS2) U8.14(CBUS3) U8.24(NC2) U8.27(OSCI) U8.28(OSCO) V1.NC V2.NC V3.NC V4.NC V5.NC V6.NC X2.4

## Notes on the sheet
- VFD Tube Clock
- ATMEGA 328P | I2C IO Expanders / VFD Drivers / VFD Tubes
- ATMEGE328P
- FT232RL USB-->UART
- USB to Serial Adaptor
- DS3231S RTC
- 1.2V Output Filament Buck
- ~25V Output Plate Boost
- Buttons
- Buzzer | Lights
- Temperature Sensor

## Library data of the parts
B1 = ruark2:BK-912
C1-C6 C8 C12-C16 C19-C21 = rcl:C-EU: CAPACITOR, European symbol
C7 C10 = rcl:C-EU: CAPACITOR, European symbol; PARTNO: 1276-1003-1-ND
C9 C11 = rcl:C-EU: CAPACITOR, European symbol; PARTNO: 490-11659-1-ND
C17 C18 = SparkFun-Passives:CAP: Capacitor
C46 = rcl:C-US: CAPACITOR, American symbol; PARTNO: 478-1682-1-ND
CR1-CR5 PWR RX TX TX6 = MySMD:LED0805
D1 D6 = diode:DIODE-: DIODE; PARTNO: RF081M2SCT-ND
JP1 = pinhead:PINHD-1X4: PIN HEADER
L1 L3 = SierraAlto:SRN4026-303M; PARTNO: SRN4026-330MCT-ND
P1 = ruark2:PKM13EPYH4000-A0
Q1-Q7 Q9 Q17-Q21 Q23-Q25 Q33-Q37 Q39-Q41 Q49-Q53 Q55-Q57 Q65-Q69 Q71-Q73 Q81-Q85 Q87-Q89 = SparkFun-DiscreteSemi:TRANSISTOR_PNP: Generic PNP BJT Double check pinouts against datasheets- not all devices are the same! MMBT3906 - 40V 200mA SOT-23 (TRANS-08052) MMBT4403 - 40V 600mA SOT-23 (TRANS-09245)
Q8 Q10-Q16 Q22 Q26-Q32 Q38 Q42-Q48 Q54 Q58-Q64 Q70 Q74-Q80 Q86 Q90-Q98 = SparkFun-DiscreteSemi:TRANSISTOR_NPN: Generic NPN BJT MMBT2222A - TRANS-08049 (SOT-23, 1A 40V) MPSA42 - TRANS-09116 (SOT-23, 500mA 300V) MMBT5088LT1G - TRANS-11160 (SOT-23, 50 mA 30V) BC547 - COM-08928 (TO-92 45V 100mA) (1.Collector 2.Base 3.Emitter) 2N3904 - COM-00521 (TO-92 40V 200mA) (1.Emitter 2.Base 3.Collector) P2N2222A -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; PROD_ID: TRANS-08049
Q99 = ruark2:MCP9700
R1-R59 R61 R74 R78-R83 = rcl:R-US_: RESISTOR, American symbol
R62 R64 = rcl:R-US_: RESISTOR, American symbol; PARTNO: 311-49.9KHRCT-ND
R63 = rcl:R-US_: RESISTOR, American symbol; PARTNO: 311-15.8KHRCT-ND
R65-R73 R75-R77 = SparkFun-Passives:RESISTOR: Resistor
R100 = ruark2:3224G-1-104E
S1 = SparkFun-Electromechanical:SWITCH-MOMENTARY-2: Various NO switches- pushbuttons, reed, etc; PROD_ID: SWCH-08441
SW1-SW6 = ruark2:EVQ-PF008K
TP3 = testpad:TP: Test pad
U1 = DS3231S:DS3231S: Extremely Accurate I2C-Integrated RTC/TCXO/Crystal; AVAILABILITY: Good; DESCRIPTION: Real Time Clock Serial 16-Pin SOIC W; MF: Maxim Integrated; MP: DS3231S#; PACKAGE: SOIC-16 Maxim Integrated; PRICE: 6.80 USD
U2-U4 = ruark2:MCP23017
U5 = SierraAlto:AOZ128CI-1; PARTNO: 785-1750-1-ND
U6 = ruark2:MIC2288
U7 = SparkFun-DigitalIC:ATMEGA328P_PDIP: uC used in the Arduino 32kb flash, 1k EEPROM, 2k SRAM This is the through-hole version of this chip.
U8 = MySMD2:FT232RL
V1-V6 = vfd:IV6_NUMITRON: Regular version with small footprint
X2 = con-hirose:MINI-USB-: MINI USB Connector Source: http://www.hirose.co.jp/cataloge_hp/e24000019.pdf; OC_FARNELL: unknown; OC_NEWARK: unknown
X3 = SierraAlto:ECS-80-20; PARTNO: XC1592CT-ND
